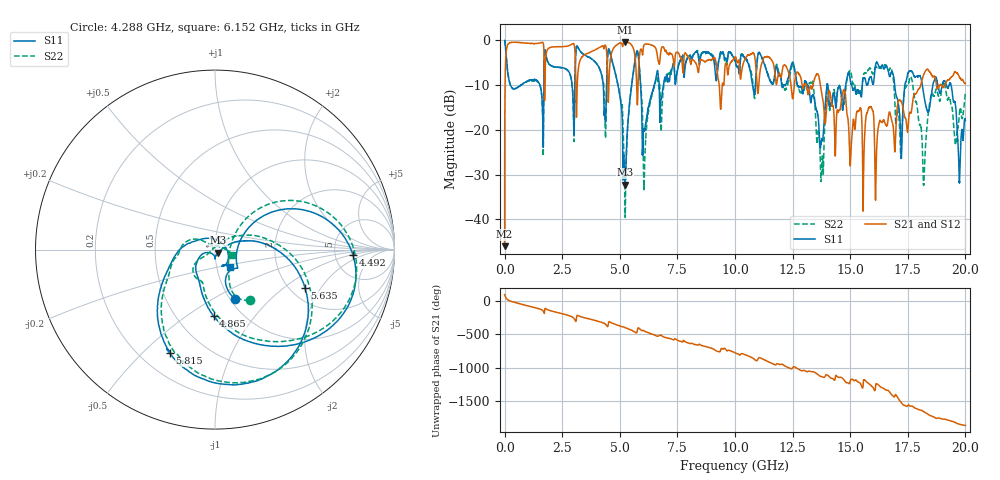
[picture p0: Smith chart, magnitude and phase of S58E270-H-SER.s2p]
!{S58E270}
!Johanson Technology Inc.
!www.johansontechnology.com
!Test Board Conditions:
!Substrate Type  RO4350B
!Substrate Thickness  60 mil
!Substrate Dk  3.66
!TL Type: GCPW
!TL Trace Width  115 mil
!TL Gap  52 mil
!Electrode orientation  Horizontal
!DUT TOPOLOGY	SERIES
!Mounting Pad LxW  55x428 mil
! Created Wed Apr 14 11:35:14 2021
# mhz S ma R 50
! 2 Port Network Data from SP1.SP block
! freq  magS11  angS11  magS21  angS21  magS12  angS12  magS22  angS22
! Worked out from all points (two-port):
!   20001 points, 300 kHz to 20 GHz, reference 50 ohm
!   highest |S21| = -0.36 dB at 5.243 GHz (marker M1); lowest = -46.0 dB at 300 kHz (marker M2)
!   |S21| within 3 dB of the highest: 56.29 MHz to 1.711 GHz (1.655 GHz wide, 187 % of centre); 1.794 GHz to 3.061 GHz (1.268 GHz wide, 52.2 % of centre)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
!   lowest |S11| = -32.3 dB at 5.23 GHz (marker M3), VSWR 1.05, Z = 51.8 - j1.68 ohm
!   |S11| at or under -10 dB: 13.14 GHz to 13.99 GHz (850.9 MHz wide, 6.27 % of centre); 14.03 GHz to 14.81 GHz (777.3 MHz wide, 5.39 % of centre); 19.38 GHz to end of sweep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
!   |S22| runs from -39.6 to 0.0 dB; largest |S21 - S12| = 0.0068
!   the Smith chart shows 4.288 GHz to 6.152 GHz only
!   S11 on the Smith chart (normalised r, x): 4.288 GHz: 1.06, -0.64; 4.492 GHz: 7.50, -1.09; 4.865 GHz: 0.75, -0.64; 5.635 GHz: 2.39, -1.45; 5.815 GHz: 0.32, -0.61; 6.152 GHz: 1.16, -0.23
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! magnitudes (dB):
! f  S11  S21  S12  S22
! 300 kHz  0.0  -46.0  -45.8  0.0
! 189.3 MHz  -8.8  -0.6  -0.6  -8.9
! 3.334 GHz  -2.7  -3.9  -3.9  -2.7
! 4.288 GHz  -10.6  -1.4  -1.4  -9.4
! 4.492 GHz  -2.3  -13.1  -13.2  -2.4
! 4.865 GHz  -8.6  -1.0  -1.0  -8.6
! 5.23 GHz  -32.3  -0.4  -0.4  -38.6
! 5.243 GHz  -31.4  -0.4  -0.4  -36.9
! 5.635 GHz  -5.3  -2.7  -2.7  -5.3
! 5.815 GHz  -4.0  -6.4  -6.5  -3.9
! 6.152 GHz  -17.8  -0.8  -0.8  -20.0
! 6.667 GHz  -7.6  -4.6  -4.6  -9.3
! 10 GHz  -4.4  -3.7  -3.7  -4.4
! 13.33 GHz  -12.5  -10.8  -10.9  -9.2
! 13.77 GHz  -22.0  -12.1  -12.1  -27.7
! 14.01 GHz  -9.7  -13.4  -13.4  -9.9
! 16.67 GHz  -7.2  -16.8  -16.9  -6.7
! 17.19 GHz  -22.3  -13.4  -13.5  -25.9
! 17.63 GHz  -6.9  -16.2  -16.4  -8.1
! 18.2 GHz  -12.3  -7.5  -7.5  -31.4
! 18.55 GHz  -11.2  -7.9  -7.9  -11.9
! 20 GHz  -17.9  -9.7  -9.6  -11.8
